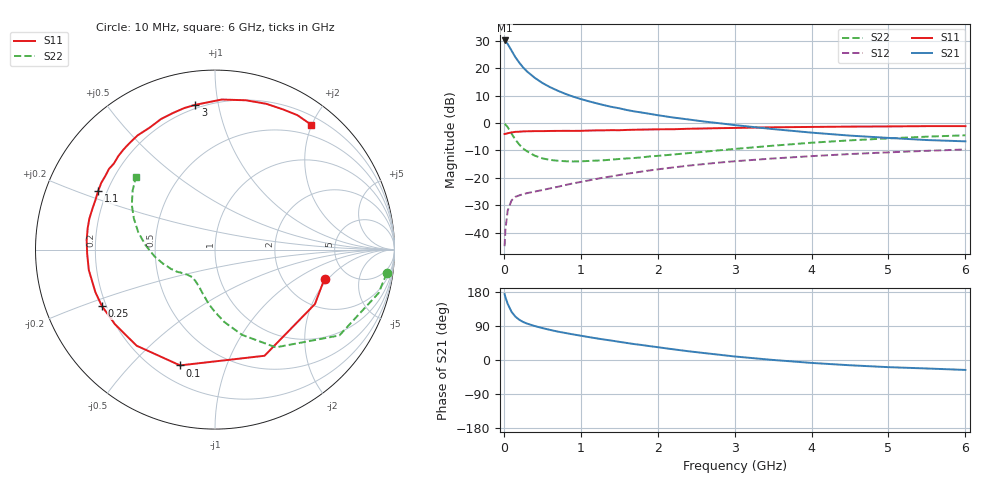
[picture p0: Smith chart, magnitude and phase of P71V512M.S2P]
! SIEMENS Small Signal Semiconductors
! BFP196
! Si NPN RF Bipolar Junction Transistor in SOT143
! VCE = 1.5 V  IC = 12 mA
! Common Emitter S-Parameters:  May  1996
# GHz  S  MA  R  50
!  f  S11  S21  S12  S22
! GHz  MAG  ANG  MAG  ANG  MAG  ANG  MAG  ANG
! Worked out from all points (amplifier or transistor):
!   36 points, 10 MHz to 6 GHz, reference 50 ohm
!   highest |S21| = 30.1 dB at 10 MHz (marker M1)
!   |S21| within 3 dB of that: start of sweep to 85.77 MHz
!   unconditionally stable (mu >= 1): 808.8 MHz to 3.421 GHz
!   at 250 MHz: K = 0.46, MSG = 23.1 dB, |S12| = -25.9 dB
!   at 1.4 GHz: K = 1.14, MAG = 10.4 dB, |S12| = -19.4 dB
!   at 6 GHz: K = 0.98, MSG = 1.5 dB, |S12| = -9.6 dB
!   S11 on the Smith chart (normalised r, x): 10 MHz: 3.37, -1.82; 100 MHz: 0.30, -0.70; 250 MHz: 0.18, -0.23; 1.1 GHz: 0.17, +0.23; 3 GHz: 0.18, +0.86; 6 GHz: 0.33, +1.99
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0.01  0.6313 -14.9  32.02 173.8  0.0057 83.5  0.9664 -7.8
0.02  0.6341 -28.6  30.77 166.0  0.0112 79.5  0.9429 -14.9
0.05  0.6527 -65.0  27.62 148.2  0.0254 62.8  0.842 -34.6
0.1  0.6739 -106.8  20.95 127.1  0.0389 47.1  0.6415 -58.1
0.15  0.6909 -129.2  15.85 114.4  0.0452 38.6  0.4984 -72.4
0.2  0.6956 -143.3  12.65 106.3  0.048 35.3  0.407 -82.6
0.25  0.7043 -153.5  10.34 100.4  0.0506 33.9  0.3441 -90.5
0.3  0.7074 -160.4  8.756 96.2  0.0527 34.0  0.3062 -96.3
0.4  0.7122 -170.8  6.705 89.7  0.0563 34.5  0.255 -105.5
0.5  0.7126 -177.9  5.384 84.3  0.0601 36.3  0.2271 -112.5
0.6  0.7171 175.7  4.513 79.5  0.0644 38.4  0.2131 -118.2
0.7  0.7194 170.3  3.889 75.0  0.0688 40.3  0.2055 -122.5
0.8  0.721 166.2  3.405 71.3  0.0742 41.5  0.2014 -126.2
1.1  0.7286 153.3  2.502 60.6  0.0898 44.3  0.2037 -134.2
1.3  0.7362 145.9  2.122 54.1  0.1018 45.1  0.21 -138.9
1.6  0.7494 136.0  1.726 44.9  0.1191 45.0  0.2265 -144.7
2.2  0.7709 118.2  1.263 28.3  0.1552 41.6  0.2669 -156.0
3  0.8141 97.7  0.919 9.3  0.2012 33.6  0.3373 -173.2
3.5  0.837 87.4  0.776 0.1  0.2261 27.9  0.3866 176.6
4.5  0.8611 70.6  0.59 -13.9  0.2724 16.8  0.4837 159.1
5.5  0.8786 58.5  0.49 -22.4  0.312 5.8  0.5645 144.4
6  0.8783 52.4  0.464 -26.2  0.3299 -0.3  0.5985 137.4
